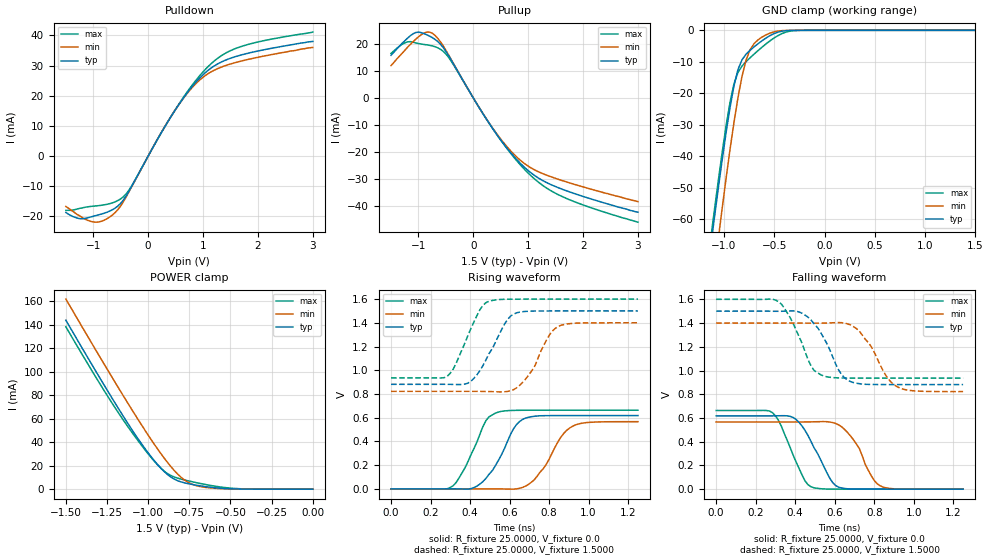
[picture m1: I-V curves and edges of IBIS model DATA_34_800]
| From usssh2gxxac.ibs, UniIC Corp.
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|When TDQS is enabled, NU_TDQS is a output with terminal resistance;
|When TDQS is disabled, NU_TDQS is a DM;
|   Model DATA_34_800
[Model]  DATA_34_800
Model_type I/O
Polarity   Non-Inverting
Enable   Active-High
Vinl =   0.60000000V
Vinh =   0.90000000V
Vmeas =   0.750000000V
Rref =   25.00000000
Vref =   0.75000000V
C_comp   1.6160pF   1.5990pF   1.6430pF
[Temperature Range]   25.0000   95.0000   0.0
[Voltage Range]   1.5000V   1.4000V   1.6000V
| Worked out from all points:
|   slope of the pulldown table from 0 to 0.225 V, typ, clamps not added: 30.8 ohm
|   slope of the pullup table from 0 to 0.225 V, typ, clamps not added: 30.4 ohm
|   GND clamp passes 1 mA (typ) near -0.50 V on its own axis
|   POWER clamp passes 1 mA (typ) near -0.58 V on its own axis
|   rising waveform, R_fixture 25.0000, V_fixture 0.0: 20-80 % time 120ps typ, 125ps min, 108ps max; typ from 0 V to 0.618 V
|   rising waveform, R_fixture 25.0000, V_fixture 1.5000: 20-80 % time 118ps typ, 111ps min, 104ps max; typ from 0.881 V to 1.5 V
|   falling waveform, R_fixture 25.0000, V_fixture 0.0: 20-80 % time 115ps typ, 107ps min, 101ps max; typ from 0.618 V to 0 V
|   falling waveform, R_fixture 25.0000, V_fixture 1.5000: 20-80 % time 115ps typ, 122ps min, 105ps max; typ from 1.5 V to 0.881 V
[Pulldown]
|Voltage   I(typ)   I(min)   I(max)
-1.5V     -18.7mA    -16.7mA    -18mA
-1.25V    -20.76mA   -19.8mA    -17.33mA
-1V       -19.96mA   -21.85mA   -16.61mA
-800mV    -18.94mA   -21.24mA   -16.16mA
-600mV    -17.23mA   -18.69mA   -15.15mA
-350mV    -11.62mA   -11.84mA   -11.29mA
200mV     6.523mA    6.58mA     6.518mA
550mV     16.83mA    16.81mA    16.97mA
850mV     24.09mA    23.66mA    24.66mA
1.15V     29.22mA    27.95mA    30.67mA
1.7V      33.54mA    31.52mA    36.35mA
3V        38mA       36mA       41.1mA
[Pullup]
|Voltage   I(typ)   I(min)   I(max)
-1.5V     15.8mA     12mA       16.5mA
-1.25V    21.14mA    17.6mA     20.39mA
-1.05V    24.23mA    21.76mA    20.4mA
-900mV    23.84mA    24.02mA    19.83mA
-750mV    22.38mA    24mA       19.29mA
-600mV    19.94mA    20.83mA    18.05mA
-450mV    15.66mA    15.92mA    15.03mA
300mV     -9.744mA   -9.622mA   -9.709mA
850mV     -24.07mA   -22.95mA   -24.6mA
1.2V      -29.82mA   -27.44mA   -31.4mA
1.55V     -33.24mA   -30.13mA   -35.83mA
3V        -42.3mA    -38.4mA    -46mA
[GND_clamp]
|Voltage   I(typ)   I(min)   I(max)
-1.5V     -169mA     -189.1mA   -163.8mA
-1.14V    -70.71mA   -88.3mA    -68.32mA
-1.1V     -60.74mA   -77.66mA   -58.33mA
-1.06V    -51.03mA   -67.22mA   -48.61mA
-1.02V    -41.65mA   -57.06mA   -39.27mA
-940mV    -24.55mA   -37.9mA    -22.88mA
-860mV    -12.39mA   -21.26mA   -13.32mA
-780mV    -7.577mA   -9.433mA   -9.942mA
-740mV    -6.329mA   -6.125mA   -8.71mA
-620mV    -3.273mA   -2.113mA   -5.305mA
-300mV    -11.81uA   -4.878uA   -91.71uA
1.5V      4.577nA    23.6nA     33.33nA
[POWER_clamp]
|Voltage   I(typ)   I(min)   I(max)
-1.5V     143.7mA    161.7mA    138.1mA
-1.22V    77.56mA    95.29mA    73.32mA
-1.12V    55.19mA    72.34mA    52.54mA
-1.02V    34.59mA    50.23mA    33.56mA
-960mV    23.77mA    37.63mA    23.28mA
-900mV    14.66mA    25.9mA     15mA
-840mV    8.415mA    15.63mA    10.28mA
-780mV    5.408mA    7.848mA    7.861mA
-700mV    3.206mA    2.693mA    5.332mA
-600mV    1.29mA     794.5uA    2.681mA
-420mV    69.47uA    44.47uA    238.7uA
0V        4.577nA    6.249nA    39.08nA
[Ramp]
| variable   typ   min   max
dV/dt_r  0.3707/0.1151n   0.3398/0.1312n   0.3978/0.1081n
dV/dt_f  0.3712/0.1121n   0.3468/0.1264n   0.3986/0.1049n
R_load = 25.0000
[Rising Waveform]
R_fixture= 25.0000
V_fixture= 0.0
V_fixture_min= 0.0
V_fixture_max= 0.0
|time   V(typ)   V(min)   V(max)
0s        0V         0V         0V
315ps     244.3uV    -1.938uV   27.18mV
435ps     23.49mV    72.13uV    395mV
480ps     87.14mV    240.9uV    573.3mV
545ps     244.2mV    -33.66uV   648.2mV
620ps     505.8mV    -2.401mV   661.4mV
680ps     595.8mV    22.19mV    662.7mV
770ps     616.7mV    168.8mV    663mV
920ps     617.9mV    528.8mV    663mV
1.25ns    617.9mV    566.4mV    663mV
[Rising Waveform]
R_fixture= 25.0000
V_fixture= 1.5000
V_fixture_min= 1.4000
V_fixture_max= 1.6000
|time   V(typ)   V(min)   V(max)
0s        881.4mV    822mV      935.7mV
285ps     881.3mV    822mV      949.9mV
405ps     908.3mV    822.1mV    1.354V
450ps     997.1mV    821.9mV    1.51V
495ps     1.137V     820.4mV    1.581V
620ps     1.473V     835.6mV    1.599V
725ps     1.499V     1.025V     1.6V
800ps     1.5V       1.292V     1.6V
845ps     1.5V       1.368V     1.6V
1.25ns    1.5V       1.4V       1.6V
[Falling Waveform]
R_fixture= 25.0000
V_fixture= 0.0
V_fixture_min= 0.0
V_fixture_max= 0.0
|time   V(typ)   V(min)   V(max)
0s        617.9mV    566.4mV    663mV
285ps     617.9mV    566.4mV    644.6mV
405ps     586.9mV    566.2mV    227.3mV
450ps     494.7mV    566.5mV    69.54mV
495ps     350mV      567.7mV    11.55mV
605ps     30.34mV    553.7mV    212.5uV
695ps     1.089mV    416.2mV    6.884uV
785ps     30uV       113.3mV    0V
830ps     5.556uV    28.24mV    0V
1.25ns    0V         703.2nV    0V
[Falling Waveform]
R_fixture= 25.0000
V_fixture= 1.5000
V_fixture_min= 1.4000
V_fixture_max= 1.6000
|time   V(typ)   V(min)   V(max)
0s        1.5V       1.4V       1.6V
315ps     1.499V     1.4V       1.581V
435ps     1.482V     1.399V     1.228V
495ps     1.395V     1.399V     1.002V
545ps     1.274V     1.4V       953.5mV
620ps     1.004V     1.404V     937.6mV
680ps     906.6mV    1.384V     936mV
770ps     883mV      1.236V     935.7mV
920ps     881.4mV    859.7mV    935.7mV
1.25ns    881.4mV    822.1mV    935.7mV
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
